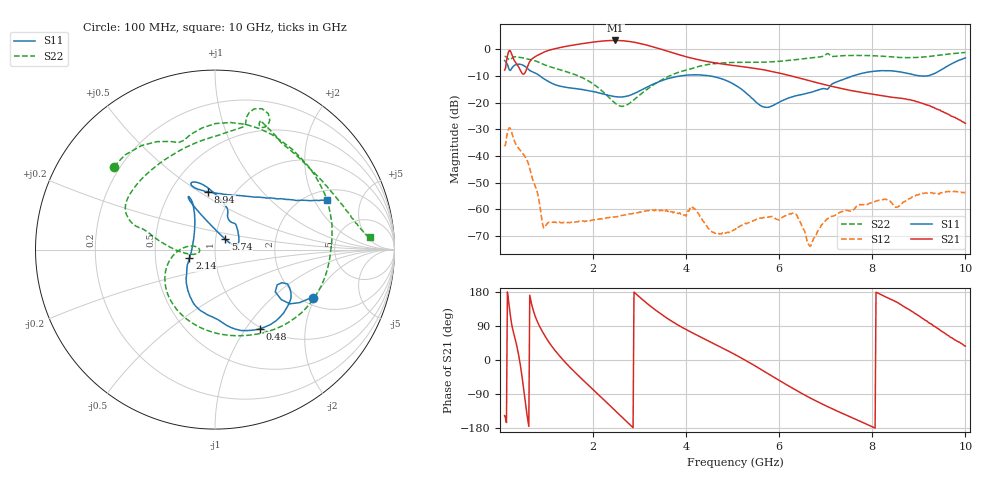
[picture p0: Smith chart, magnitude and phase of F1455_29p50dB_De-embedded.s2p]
! Integrated Device Technology
! Corporate Headquarters
! 6024 Silver Creek Valley Road
! San Jose, CA 95138  USA
! Phone:  1-408-284-8200
! Toll Free:  1-800-223-1366
! Webpage:  http://www.idt.com/
! Timing and RF Division
! 515 Groton Road, Suite 102
! Westford, MA 01886-6024
! Device:  F1455
! Description: 6-bit 0.5 dB Transmit Variable Gain Amplifier
! Frequency:  1400.0 -  2300.00 MHz
! Package:  6x6 mm Thin QFN Plastic Package: 28 pin
! State:  59
! Atten State:  29.5 dB
! Voltage:  +5.00 Volts
! Current:  217.605 mA
! Data:  The device was measured on a the F1455 evaluation board which has
!  individual transmission lines to the RF pins.  Data was collected
!  using a calibrated network analyzer.  The evaluation board was
!  de-embedded using a TRL calibration technique.
!  The reference plane is the edge of the package pin.
!  Pin  1 = CSb
!  Pin  2 = DATA
!  Pin  3 = CLK
!  Pin  4 = RSET
!  Pin  5 = GND
!  Pin  6 = RFIN  = Port 1
!  Pin  7 = GND
!  Pin  8 = NC
!  Pin  9 = NC
!  Pin 10 = NC
!  Pin 11 = NC
!  Pin 12 = NC
!  Pin 13 = NC
!  Pin 14 = /STBY
!  Pin 15 = GND
!  Pin 16 = RFOUT  = Port 2
!  Pin 17 = GND
!  Pin 18 = NC
!  Pin 19 = NC
!  Pin 20 = NC
!  Pin 21 = GND
!  Pin 22 = NC
!  Pin 23 = GND
!  Pin 24 = NC
!  Pin 25 = NC
!  Pin 26 = NC
!  Pin 27 = GND
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# GHz S dB R 50
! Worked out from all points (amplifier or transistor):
!   496 points, 100 MHz to 10 GHz, reference 50 ohm
!   highest |S21| = 3.2 dB at 2.48 GHz (marker M1)
!   |S21| within 3 dB of that: 1.202 GHz to 3.41 GHz (2.208 GHz wide, 95.8 % of centre)
!   unconditionally stable (mu >= 1): start of sweep to end of sweep
!   at 1.74 GHz: K = 574.67, MAG = 2.5 dB, |S12| = -64.3 dB
!   at 5.06 GHz: K = 1569.10, MAG = -4.4 dB, |S12| = -67.4 dB
!   at 10 GHz: K = 793.61, MAG = -19.1 dB, |S12| = -53.7 dB
!   S11 on the Smith chart (normalised r, x): 100 MHz: 2.27, -1.94; 480 MHz: 0.98, -1.16; 2.14 GHz: 0.75, -0.07; 5.74 GHz: 1.11, +0.13; 8.94 GHz: 0.76, +0.54; 10 GHz: 2.43, +2.56
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0.1  -4.29 -26.1  -7.87 -146.5  -36.38 47.8  -2.74 140.7
0.18  -6.70 -37.0  -1.24 161.6  -30.08 -6.3  -3.72 112.4
0.26  -7.00 -25.3  -2.24 89.2  -31.60 -77.4  -3.33 96.1
0.38  -5.67 -42.7  -6.04 26.9  -36.64 -118.8  -2.99 58.2
0.48  -5.89 -60.7  -9.14 -48.9  -38.84 -150.6  -3.24 31.7
0.66  -8.19 -87.8  -4.18 158.4  -46.07 139.6  -3.93 -10.1
0.96  -11.28 -123.6  -1.02 64.8  -66.66 131.3  -5.89 -70.5
1.34  -14.04 -142.4  0.77 2.3  -64.95 121.6  -7.98 -121.0
1.76  -15.10 -151.2  2.03 -50.2  -64.34 93.6  -10.61 -157.9
2.14  -16.43 -161.1  2.92 -94.2  -63.50 78.5  -14.83 177.7
2.48  -17.82 178.3  3.24 -134.4  -62.73 69.2  -20.31 173.3
2.86  -16.81 143.3  2.64 -178.6  -61.52 58.8  -19.21 -167.1
3.4  -12.28 118.6  0.30 126.6  -60.09 36.8  -12.30 177.6
4.1  -9.65 116.2  -3.30 73.9  -59.34 16.9  -7.39 163.9
5.06  -13.48 111.8  -6.23 13.6  -67.44 44.4  -4.96 148.8
5.74  -21.81 45.0  -7.98 -34.7  -62.86 34.8  -4.84 120.5
6.34  -17.54 14.0  -10.41 -78.2  -61.66 -9.7  -3.99 89.8
6.7  -16.10 34.3  -12.06 -102.3  -72.46 -178.3  -3.25 78.9
7.1  -13.65 70.3  -13.83 -126.5  -62.93 107.6  -2.43 67.0
8.36  -8.08 109.5  -17.83 162.3  -56.67 63.5  -2.82 62.9
8.94  -9.78 97.0  -19.65 121.4  -54.62 74.1  -3.14 39.3
10  -3.29 24.0  -27.81 36.8  -53.66 7.0  -1.26 4.7
